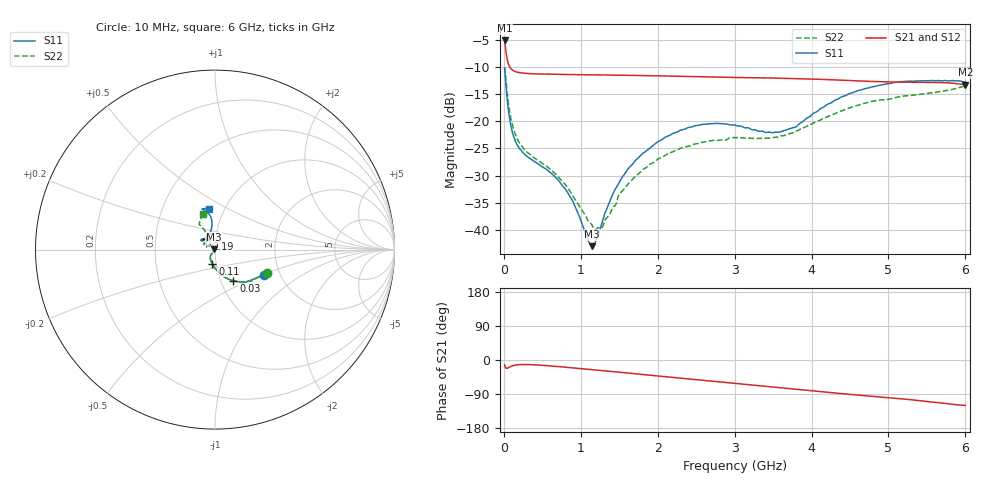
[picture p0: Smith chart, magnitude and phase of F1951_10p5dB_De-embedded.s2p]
! Integrated Device Technology
! Corporate Headquarters
! 6024 Silver Creek Valley Road
! San Jose, CA 95138  USA
! Phone:  1-408-284-8200
! Toll Free:  1-800-223-1366
! Webpage:  http://www.idt.com/
! Timing and RF Division
! 515 Groton Road, Suite 102
! Westford, MA 01886-6024
! Device:  F1951
! Description: 6-bit 0.5 dB Digital Step Attenuator
! Frequency:  100.0 -  4000.00 MHz
! Package:  4x4 mm Thin QFN Plastic Package: 24 pin
! Ports:  2 RF, 6 DC
!  Pin  1  = NC
!  Pin  2  = RF1  =  Port 1
!  Pin  3  = GND
!  Pin  4  = NC
!  Pin  5  = Serial Data Out (SDO)
!  Pin  6  = NC
!  Pin  7  = Reset Bar ( RSTb)
!  Pin  8  = Clock (CLK)
!  Pin  9  = Chip Select Bar (CSb)
!  Pin 10  = NC
!  Pin 11  = Serial Data In (SDI)
!  Pin 12  = NC
!  Pin 13  = NC
!  Pin 14  = VDD
!  Pin 15  = NC
!  Pin 16  = GND
!  Pin 17  = RF2  =  Port 2
!  Pin 18  = NC
!  Pin 19  = GND
!  Pin 20  = GND
!  Pin 21  = GND
!  Pin 22  = GND
!  Pin 23  = GND
!  Pin 24  = GND
! State:  21
! Atten State:  10.5 dB
! Voltage:  +3.30 Volts
! Current:  0.488 mA
! Data:  The device was measured on a F195X evaluation board which has
!  individual transmission lines to the RF pins.  Data was collected
!  de-embedded using a Automatic Fixture Removal [AFR] (Keysight Technologies).
!  The reference plane is the edge of the package pin.
! Misc:  Lot Code  1225BCA
!  Action Tracker AT0399
! Date Measured:  2018-09-13
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# GHz S dB R 50
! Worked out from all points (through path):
!   600 points, 10 MHz to 6 GHz, reference 50 ohm
!   highest |S21| = -5.14 dB at 10 MHz (marker M1); lowest = -13.3 dB at 6 GHz (marker M2)
!   group delay of S21, straight-line fit = 52.4 ps
!   lowest |S11| = -43.0 dB at 1.15 GHz (marker M3), VSWR 1.01, Z = 49.3 + j0.0566 ohm
!   |S11| at or under -10 dB: start of sweep to end of sweep
!   |S22| runs from -40.0 to -10.0 dB; largest |S21 - S12| = 0.00046
!   S11 on the Smith chart (normalised r, x): 10 MHz: 1.64, -0.52; 30 MHz: 1.15, -0.42; 110 MHz: 0.96, -0.15; 2.19 GHz: 0.90, +0.11; 6 GHz: 0.85, +0.41
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0.01  -10.27 -27.8  -5.14 -13.0  -5.14 -13.0  -10.02 -24.3
0.03  -13.83 -59.8  -7.47 -21.8  -7.47 -21.8  -12.98 -53.6
0.07  -19.07 -86.8  -9.82 -19.0  -9.82 -19.0  -17.75 -81.3
0.11  -21.99 -100.2  -10.57 -15.4  -10.57 -15.4  -20.61 -95.5
0.17  -24.25 -112.3  -10.96 -12.9  -10.96 -12.9  -23.13 -108.4
0.27  -26.07 -121.9  -11.18 -11.9  -11.18 -11.9  -25.30 -119.9
0.8  -32.49 -126.0  -11.39 -19.0  -11.39 -19.0  -31.66 -130.2
1.01  -38.59 -135.6  -11.45 -22.8  -11.45 -22.8  -36.31 -137.4
1.15  -42.97 175.4  -11.46 -25.4  -11.46 -25.4  -39.18 -160.4
1.27  -38.98 128.2  -11.48 -27.7  -11.48 -27.7  -39.66 165.6
1.4  -33.94 114.9  -11.51 -30.2  -11.51 -30.2  -36.38 140.1
1.53  -30.47 113.7  -11.53 -32.7  -11.54 -32.7  -32.97 131.3
1.73  -26.93 116.6  -11.57 -36.7  -11.58 -36.7  -29.88 129.3
2.01  -23.71 124.5  -11.65 -42.3  -11.65 -42.3  -26.90 134.3
2.19  -22.29 129.4  -11.71 -45.9  -11.71 -45.9  -25.64 138.7
2.58  -20.58 140.3  -11.82 -53.7  -11.82 -53.6  -23.84 148.3
3.01  -20.72 146.7  -11.95 -62.0  -11.95 -62.0  -22.97 152.0
3.58  -21.99 123.6  -12.07 -73.1  -12.07 -73.1  -22.78 134.1
4.01  -18.72 99.9  -12.23 -81.5  -12.23 -81.5  -20.46 120.6
4.49  -14.92 97.0  -12.51 -90.5  -12.51 -90.5  -17.57 119.2
5.01  -13.08 104.4  -12.78 -99.6  -12.78 -99.6  -15.95 121.9
6  -12.77 98.4  -13.29 -119.8  -13.29 -119.8  -13.51 108.2
